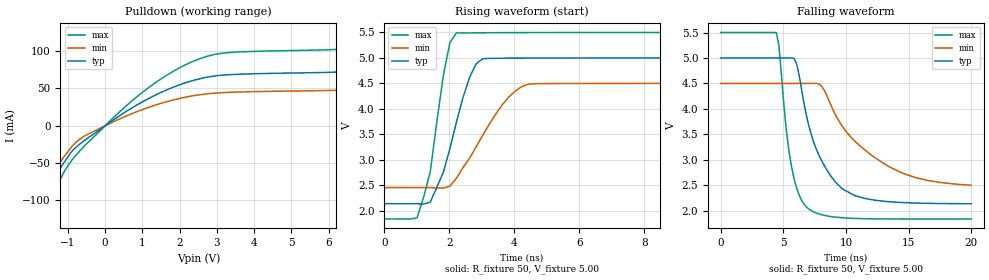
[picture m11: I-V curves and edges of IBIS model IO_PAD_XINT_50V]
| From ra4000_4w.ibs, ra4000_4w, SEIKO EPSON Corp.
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[Model]   IO_PAD_XINT_50V
Model_type Open_drain
Polarity Non-Inverting
Vref=5.50
Vmeas=2.50
Rref=5000
C_comp   2.5p   2.0p   3.0p
[Temperature Range] 25   125   -40
[Voltage Range]   5.00   4.50   5.50
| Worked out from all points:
|   slope of the pulldown table from 0 to 0.75 V, typ, clamps not added: 30.2 ohm
|   falling waveform, R_fixture 50, V_fixture 5.00: 20-80 % time 2.29ns typ, 4.45ns min, 1.11ns max; typ from 5 V to 2.14 V
|   rising waveform, R_fixture 50, V_fixture 5.00: 20-80 % time 741ps typ, 1.2ns min, 517ps max; typ from 2.14 V to 5 V
[Pulldown]
-5V       -520.2mA   -422.2mA   -640.6mA
-2.1V     -150.2mA   -131.1mA   -176.6mA
-2V       -137.7mA   -121.4mA   -161.3mA
-1.8V     -113.5mA   -101.8mA   -136.1mA
-1.1V     -48.86mA   -41.26mA   -61.43mA
-600mV    -21.34mA   -14.99mA   -29.25mA
1.1V      34.77mA    23.54mA    48.65mA
2.6V      63.75mA    42.01mA    90.93mA
3.3V      68.39mA    44.77mA    98.05mA
7.4V      77.39mA    51.54mA    109.5mA
8.8V      96.9mA     65.68mA    135.2mA
10V       126.3mA    87.31mA    173.8mA
[Falling Waveform]
R_fixture=50
V_fixture=5.00
V_fixture_min=4.50
V_fixture_max=5.50
0s        5V         4.5V       5.5V
4.444ns   5V         4.5V       5.496V
4.646ns   5V         4.5V       5.257V
5.657ns   5.002V     4.5V       2.87V
6.061ns   4.891V     4.5V       2.449V
7.071ns   3.639V     4.5V       2.029V
8.687ns   2.721V     4.139V     1.891V
10.71ns   2.297V     3.368V     1.85V
14.55ns   2.161V     2.736V     1.838V
20ns      2.138V     2.501V     1.837V
[Rising Waveform]
R_fixture=50
V_fixture=5.00
V_fixture_min=4.50
V_fixture_max=5.50
0s        2.136V     2.452V     1.837V
1.01ns    2.135V     2.453V     1.862V
1.414ns   2.166V     2.452V     2.758V
1.818ns   2.754V     2.444V     4.654V
2.02ns    3.222V     2.482V     5.301V
2.222ns   3.741V     2.639V     5.493V
2.828ns   4.887V     3.255V     5.493V
3.636ns   4.994V     4.085V     5.496V
4.444ns   4.997V     4.487V     5.497V
20ns      5V         4.5V       5.5V
[Ramp]
R_load=50
dV/dt_r   1.719E+0/7.274E-10   1.229E+0/1.200E-9   2.198E+0/4.900E-10
dV/dt_f   1.717E+0/2.290E-9   1.199E+0/4.455E-9   2.198E+0/1.097E-9
|[End   IO_PAD_XINT_50V
